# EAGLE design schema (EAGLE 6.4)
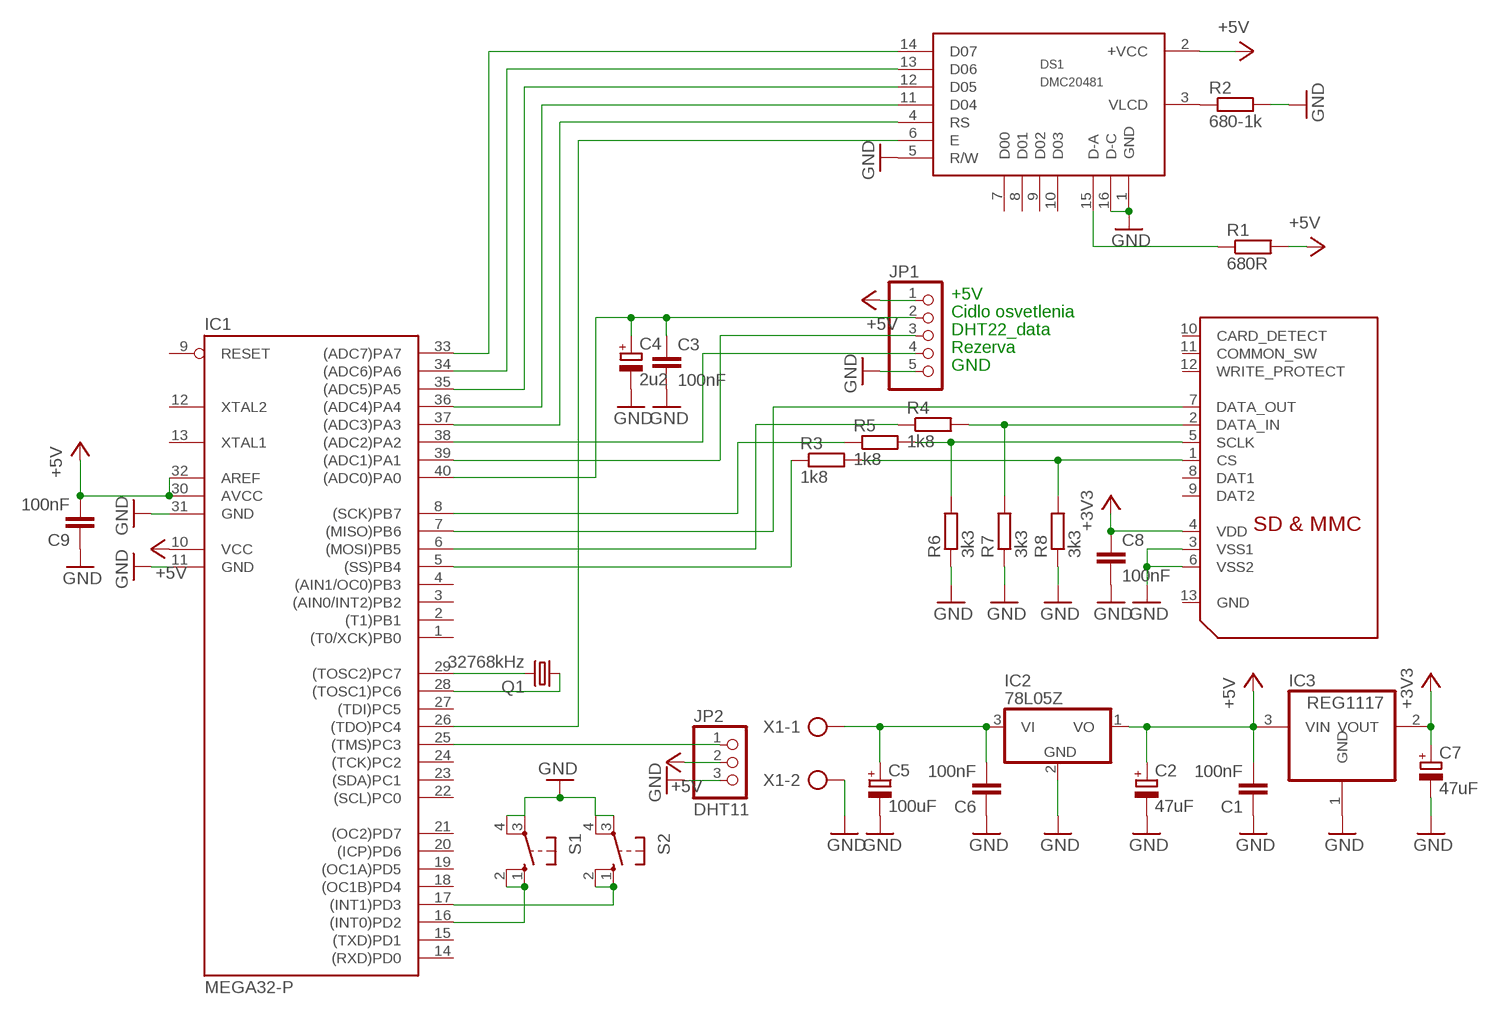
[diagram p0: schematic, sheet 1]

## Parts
C1  100nF  C-EU050-024X044  [C050-024X044]
C2  47uF  CPOL-EUE2.5-5  [E2,5-5]
C3  100nF  C-EU050-024X044  [C050-024X044]
C4  2u2  CPOL-EUE2.5-5  [E2,5-5]
C5  100uF  CPOL-EUE2.5-5  [E2,5-5]
C6  100nF  C-EU050-024X044  [C050-024X044]
C7  47uF  CPOL-EUE2.5-5  [E2,5-5]
C8  100nF  C-EU050-024X044  [C050-024X044]
C9  100nF  C-EU050-024X044  [C050-024X044]
DS1  DMC20481  [DM20481]
IC1  MEGA32-P  [DIL40]
IC2  78L05Z  [TO92]
IC3  REG1117  [SOT223]
JP1  PINHD-1X5  [1X05]
JP2  DHT11  PINHD-1X3  [1X03]
Q1  32768kHz  CRYSTALTC26V  [TC26V]
R1  680R  R-EU_0207/10  [0207/10]
R2  680-1k  R-EU_0207/10  [0207/10]
R3  1k8  R-EU_0207/10  [0207/10]
R4  1k8  R-EU_0207/10  [0207/10]
R5  1k8  R-EU_0207/10  [0207/10]
R6  3k3  R-EU_0207/10  [0207/10]
R7  3k3  R-EU_0207/10  [0207/10]
R8  3k3  R-EU_0207/10  [0207/10]
S1  10-XX  [B3F-10XX]
S2  10-XX  [B3F-10XX]
U$1  SDMMCSCDA  [SCDA]
X1  AK500/2  [AK500/2]

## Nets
+3V3: C7.+ C8.1 IC3.2(VOUT) U$1.4(VDD)
+5V: C1.2 C2.+ C9.2 DS1.2(+VCC) IC1.10(VCC) IC1.30(AVCC) IC1.32(AREF) IC2.1(VO) IC3.3(VIN) JP1.1 JP2.2 R1.2
GND: C1.1 C2.- C3.2 C4.- C5.- C6.1 C7.- C8.2 C9.1 DS1.1(GND) DS1.5(R/W) DS1.16(D-C) IC1.11(GND) IC1.31(GND) IC2.2(GND) IC3.1(GND) JP1.5 JP2.3 R2.2 R6.1 R7.1 R8.1 S1.3(P) S1.4(P1) S2.3(P) S2.4(P1) U$1.3(VSS1) U$1.6(VSS2) X1.2
N$1: IC1.28((TOSC1)PC6) Q1.1
N$2: IC1.29((TOSC2)PC7) Q1.2
N$3: C3.1 C4.+ IC1.40((ADC0)PA0) JP1.2
N$4: IC1.39((ADC1)PA1) JP1.3
N$5: IC1.38((ADC2)PA2) JP1.4
N$6: DS1.11(D04) IC1.36((ADC4)PA4)
N$7: DS1.12(D05) IC1.35((ADC5)PA5)
N$8: DS1.13(D06) IC1.34((ADC6)PA6)
N$9: DS1.14(D07) IC1.33((ADC7)PA7)
N$10: DS1.15(D-A) R1.1
N$11: DS1.3(VLCD) R2.1
N$13: DS1.4(RS) IC1.37((ADC3)PA3)
N$15: C5.+ C6.2 IC2.3(VI) X1.1
N$16: R5.2 R6.2 U$1.5(SCLK)
N$17: IC1.16((INT0)PD2) S1.1(S) S1.2(S1)
N$18: IC1.17((INT1)PD3) S2.1(S) S2.2(S1)
N$19: IC1.25((TMS)PC3) JP2.1
N$20: IC1.5((SS)PB4) R3.1
N$21: IC1.6((MOSI)PB5) R4.1
N$22: IC1.7((MISO)PB6) U$1.7(DATA_OUT)
N$23: IC1.8((SCK)PB7) R5.1
N$24: R4.2 R7.2 U$1.2(DATA_IN)
N$25: R3.2 R8.2 U$1.1(CS)
N$66: DS1.6(E) IC1.26((TDO)PC4)
Unconnected: DS1.7(D00) DS1.8(D01) DS1.9(D02) DS1.10(D03) IC1.1((T0/XCK)PB0) IC1.2((T1)PB1) IC1.3((AIN0/INT2)PB2) IC1.4((AIN1/OC0)PB3) IC1.9(RESET) IC1.12(XTAL2) IC1.13(XTAL1) IC1.14((RXD)PD0) IC1.15((TXD)PD1) IC1.18((OC1B)PD4) IC1.19((OC1A)PD5) IC1.20((ICP)PD6) IC1.21((OC2)PD7) IC1.22((SCL)PC0) IC1.23((SDA)PC1) IC1.24((TCK)PC2) IC1.27((TDI)PC5) U$1.8(DAT1) U$1.9(DAT2) U$1.10(CARD_DETECT) U$1.11(COMMON_SW) U$1.12(WRITE_PROTECT) U$1.13(GND)

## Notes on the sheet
- +5V
- Cidlo osvetlenia
- DHT22_data
- Rezerva
- GND

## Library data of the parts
C1 C3 C6 C8 C9 = rcl:C-EU: CAPACITOR, European symbol
C2 C4 C5 C7 = rcl:CPOL-EU: POLARIZED CAPACITOR, European symbol
DS1 = abi-lcd:DMC20481
IC1 = atmel:MEGA32-P: MICROCONTROLLER 32 Kbytes FLASH 2 Kbytes SRAM 1 Kbytes EEPROM USART 8-channel 10 bit ADC Source: www.atmel.com .. doc2503.pdf; MPN: ATMEGA32-16PU; OC_FARNELL: 1661729; OC_NEWARK: 51P1794
IC2 = linear:78*: Positive VOLTAGE REGULATOR Source: http://cache.national.com/ds/LM/LM78L05.pdf http://www.fairchildsemi.com/ds/LM/LM7805.pdf
IC3 = burr-brown:REG1117: 800mA and 1A Low Dropout (LDO) Positive Regulator 1.8V, 2.5V, 2.85V, 3.3V, 5V, and Adj; MPN: REG1117; OC_FARNELL: 1097566; OC_NEWARK: 14P6981
JP1 = pinhead:PINHD-1X5: PIN HEADER
JP2 = pinhead:PINHD-1X3: PIN HEADER
Q1 = crystal:CRYSTAL: CRYSTAL; OC_FARNELL: unknown; OC_NEWARK: unknown
R1-R8 = rcl:R-EU_: RESISTOR, European symbol
S1 S2 = switch-omron:10-XX: OMRON SWITCH; MPN: B3F-1000; OC_FARNELL: 176432; OC_NEWARK: 36M3542
U$1 = adafruit:SDMMC: SD MMC Card holder 4UCON part #06132 - easy to solder
X1 = con-ptr500:AK500/2: CONNECTOR; OC_FARNELL: unknown; OC_NEWARK: unknown

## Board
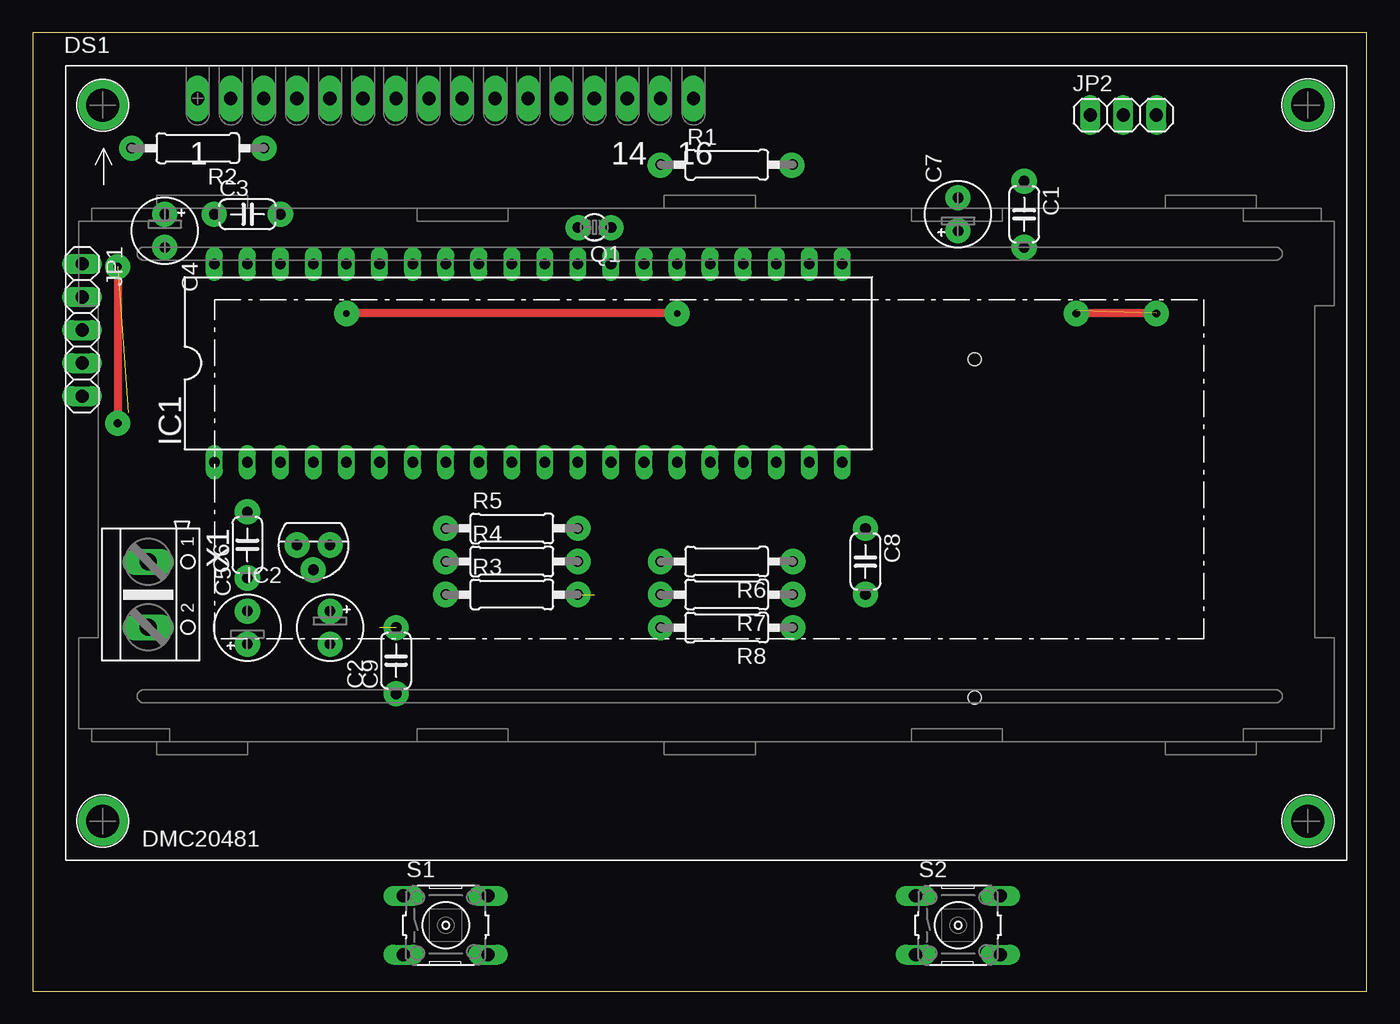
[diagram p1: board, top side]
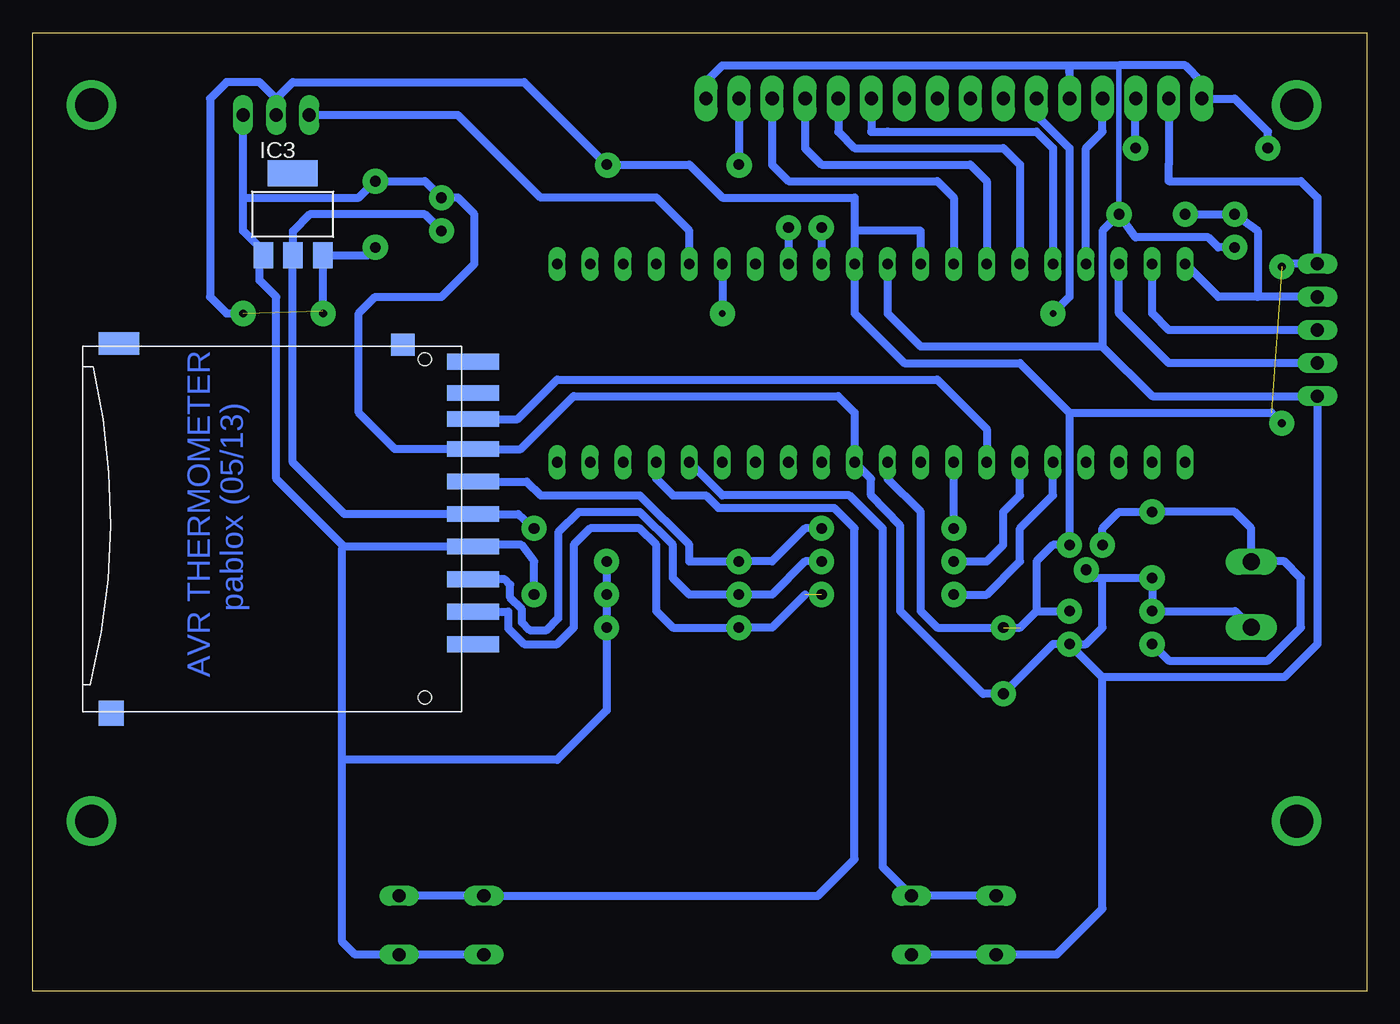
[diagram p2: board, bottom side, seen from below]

Size 102.54 x 73.65 mm. Coordinates in mm from the lower left corner, seen from the top.
Outline: 0,0 102.54,0 102.54,73.65 0,73.65 0,0
Copper layers (1*16): Top 0.035mm / dielectric 1.5mm / Bottom 0.035mm
Design rules "default": minimum track width 10mil, minimum drill 24mil, track to track 8mil, track to pad 8mil, pad to pad 8mil, via to via 8mil, smd to smd 8mil, copper to edge 40mil, drill to drill 8mil, minimum pad ring 10mil, minimum via ring 8mil, stop-mask expansion 4mil, vias tented up to drill 0mil, thermal gap 10mil

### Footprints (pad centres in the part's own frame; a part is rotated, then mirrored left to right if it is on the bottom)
C050-024X044 = drill 0.813 octagon: 1 -2.54,0; 2 2.54,0
E2,5-5 = drill 0.813 pad 1.6: + -1.27,0 | drill 0.813 pad 1.6 octagon: - 1.27,0
DM20481 = drill 1.016 pad 1.778 long: 1 -39.383,29.21; 2 -36.843,29.21; 3 -34.303,29.21; 4 -31.763,29.21; 5 -29.223,29.21; 6 -26.683,29.21; 7 -24.143,29.21; 8 -21.603,29.21; 9 -19.063,29.21; 10 -16.523,29.21; 11 -13.983,29.21; 12 -11.443,29.21; 13 -8.903,29.21; 14 -6.363,29.21; 15 -3.823,29.21; 16 -1.283,29.21 | drill 2.54 pad 3.81: P$1 -46.672,-26.289; P$2 45.936,-26.289; P$3 45.936,28.715; P$4 -46.672,28.702
DIL40 = drill 0.813 long: 1 -24.13,-7.62; 2 -21.59,-7.62; 3 -19.05,-7.62; 4 -16.51,-7.62; 5 -13.97,-7.62; 6 -11.43,-7.62; 7 -8.89,-7.62; 8 -6.35,-7.62; 9 -3.81,-7.62; 10 -1.27,-7.62; 11 1.27,-7.62; 12 3.81,-7.62; 13 6.35,-7.62; 14 8.89,-7.62; 15 11.43,-7.62; 16 13.97,-7.62; 17 16.51,-7.62; 18 19.05,-7.62; 19 21.59,-7.62; 20 24.13,-7.62; 21 24.13,7.62; 22 21.59,7.62; 23 19.05,7.62; 24 16.51,7.62; 25 13.97,7.62; 26 11.43,7.62; 27 8.89,7.62; 28 6.35,7.62; 29 3.81,7.62; 30 1.27,7.62; 31 -1.27,7.62; 32 -3.81,7.62; 33 -6.35,7.62; 34 -8.89,7.62; 35 -11.43,7.62; 36 -13.97,7.62; 37 -16.51,7.62; 38 -19.05,7.62; 39 -21.59,7.62; 40 -24.13,7.62
TO92 = drill 0.813 octagon: 1 -1.27,0; 2 0,1.905; 3 1.27,0
SOT223 = smd 1.499 x 2.007: 1 -2.261,-3.15; 2 0.025,-3.15; 3 2.311,-3.15 | smd 3.81 x 2.007: 4 0,3.15
1X05 = drill 1.016 long: 1 -5.08,0; 2 -2.54,0; 3 0,0; 4 2.54,0; 5 5.08,0
1X03 = drill 1.016 long: 1 -2.54,0; 2 0,0; 3 2.54,0
TC26V = drill 0.813: 1 -1.27,0; 2 1.27,0
0207/10 = drill 0.813 octagon: 1 -5.08,0; 2 5.08,0
B3F-10XX = drill 1.016 long: 1 -3.251,2.261; 2 3.251,2.261; 3 -3.251,-2.261; 4 3.251,-2.261
SCDA = smd 1.2 x 4: 1 6.4,3.7; 2 3.9,3.7; 3 1.4,3.7; 4 -1.1,3.7; 5 -3.6,3.7; 6 -6.1,3.7; 7 -8.4,3.7; 8 -10.4,3.7; 9 8.9,3.7; 10 -12.8,3.7 | smd 1.7 x 1.8: 11 -14.1,-1.7 | smd 1.7 x 3.1: 12 -14.2,-23.5 | smd 1.9 x 1.9: 13 14.2,-24.1 | hole 1: -13,0; 13,0
AK500/2 = drill 1.321 long: 1 -2.515,0; 2 2.515,0

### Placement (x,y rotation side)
C1  76.2,59.69 270 top
C2  22.86,27.94 270 top
C3  16.51,59.69 0 top
C4  10.16,58.42 270 top
C5  16.51,27.94 90 top
C6  16.51,34.29 90 top
C7  71.12,59.69 90 top
C8  64,33.02 270 top
C9  27.94,25.4 90 top
DS1  52.07,39.37 0 top
IC1  38.1,48.26 0 top
IC2  21.59,34.29 180 top
IC3  82.55,59.69 0 bottom
JP1  3.81,50.8 270 top
JP2  83.82,67.31 0 top
Q1  43.18,58.69 180 top
R1  53.34,63.5 0 top
R2  12.7,64.77 180 top
R3  36.83,30.48 0 top
R4  36.83,33.02 0 top
R5  36.83,35.56 0 top
R6  53.34,33.02 180 top
R7  53.34,30.48 180 top
R8  53.34,27.94 180 top
S1  31.75,5.08 0 top
S2  71.12,5.08 0 top
U$1  72.39,35.56 270 bottom
X1  8.89,30.48 270 top

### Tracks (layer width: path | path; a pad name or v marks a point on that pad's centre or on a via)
+3V3
  Bottom 0.61: C7.+ 72.39,59.69 81.23,59.69 82.53,58.4 IC3.2 82.55,56.52 82.55,40.64 78.57,36.66 U$1.4 65.2,36.66 C8.1
+5V  (3 unrouted)
  Bottom 0.61: 39.37,58.42 39.37,60.96 49.53,60.96 52.07,63.5 R1.2 64.77,69.85 82.55,69.85 83.82,68.58 | 39.37,58.42 IC1.30 39.37,52.07 35.56,48.26 26.67,48.26 22.86,44.45 | DS1.2 15.23,63.51 15.24,62.23 5.08,62.23 3.81,60.96 JP1.1 6.31,55.88 6.54,55.65 | C1.2 76.81,56.54 IC3.3 80.24,52.3 80.21,52.07 | 25.4,29.21 26.67,27.94 33.02,27.94 34.29,29.21 34.29,36.83 36.83,39.37 IC1.10 | 25.4,29.21 C2.+ | IC1.32 34.29,58.42 39.37,58.42 | 22.86,44.45 IC2.1 24.13,34.29 25.4,33.02 25.4,29.21 | 22.86,44.45 7.34,44.45 6.54,43.65 | JP2.2 83.82,68.58 | 83.82,68.58 85.09,69.85 87.63,69.85 88.9,68.58 88.9,53.34 87.63,52.07 86.36,52.07
GND
  Bottom 0.406: 19.05,71.12 C3.2
  Bottom 0.61: 22.85,69.86 DS1.5 22.85,70.84 22.84,70.85 22.84,71.1 22.86,71.12 | 22.85,69.86 22.86,71.12 | 12.7,68.59 12.7,69.85 13.97,71.12 19.05,71.12 22.86,71.12 | 12.7,68.59 DS1.1 | DS1.1 10.16,68.58 7.62,66.04 R2.2 | DS1.16 50.79,69.86 49.53,71.12 22.86,71.12 | X1.2 10.13,29.21 C5.- C6.1 20.32,31.75 | 20.32,31.75 20.95,31.75 IC2.2 | C2.- 21.59,26.67 20.32,27.94 20.32,31.75 | R7.1 R8.1 58.42,25.4 | 20.32,24.13 6.35,24.13 3.81,26.67 JP1.5 16.51,45.72 20.32,49.53 | 20.32,24.13 C2.- | U$1.3 68.69,34.18 68.58,34.29 | C4.- 11.43,57.15 12.2,57.92 17.78,57.92 C3.2 20.32,58.42 20.32,49.53 | DS1.1 12.7,68.59 | 22.85,69.86 22.86,69.85 | IC1.31 36.83,52.07 34.29,49.53 20.32,49.53 | 86.36,60.96 JP2.3 | 86.36,60.96 86.36,58.42 84.81,56.87 IC3.1 85.09,56.26 85.09,54.61 83.82,53.34 83.82,39.37 78.61,34.16 | 86.36,60.96 77.47,60.96 C1.1 72.39,62.23 C7.- 69.85,60.96 68.58,59.69 68.58,55.88 71.12,53.34 76.2,53.34 77.47,52.07 77.47,44.45 74.68,41.66 U$1.6 65.02,41.66 60.96,45.72 40.64,45.72 39.37,44.45 IC1.11 38.1,39.37 38.1,38.1 35.86,35.76 35.86,29.21 29.51,22.86 C9.1 24.13,26.67 C2.- | 20.32,24.13 20.32,6.35 23.85,2.82 S1.3 S1.4 | U$1.3 78.61,34.16 | R6.1 R7.1 | C8.2 64,33.02 64.97,34.29 68.56,34.29 U$1.3 | S2.3 S2.4 77.75,2.82 78.74,3.81 78.74,17.78 | 78.74,17.78 62.23,17.78 58.42,21.59 R7.1 | 78.74,17.78 78.74,34.03 78.61,34.16
N$1
  Bottom 0.61: Q1.1 IC1.28
N$2
  Bottom 0.61: Q1.2 IC1.29
N$3
  Bottom 0.61: JP1.2 8.39,53.34 | 8.39,53.34 11.43,53.34 IC1.40 | C3.1 C4.+ 8.39,58.42 8.39,53.34
N$4
  Bottom 0.61: JP1.3 15.24,50.8 16.51,52.07 IC1.39
N$5
  Bottom 0.61: JP1.4 15.24,48.26 19.05,52.07 IC1.38
N$6
  Bottom 0.61: DS1.11 38.09,66.05 | 38.09,66.05 38.1,66.04 | 38.09,66.05 38.09,66.03 36.83,66.04 25.4,66.04 24.13,64.77 IC1.36
N$7
  Bottom 0.61: DS1.12 40.63,66.03 39.37,64.77 27.94,64.77 26.67,63.5 IC1.35
N$8
  Bottom 0.61: DS1.13 43.17,64.76 41.91,63.5 30.48,63.5 29.21,62.23 IC1.34
N$9
  Bottom 0.61: DS1.14 45.71,63.49 44.45,62.23 33.02,62.23 31.75,60.96 IC1.33
N$10
  Bottom 0.61: DS1.15 48.25,63.51 R1.1
N$11
  Bottom 0.61: R2.1 17.78,68.57 DS1.3
N$12  (via drill 0.6 pad 1.93)
  Top 0.61: v6.54,55.65 v6.54,43.65
N$13
  Bottom 0.61: IC1.37 21.59,64.77 20.32,66.04 20.32,68.57 DS1.4
N$15
  Bottom 0.61: IC2.3 20.32,35.56 19.05,36.83 C6.2 10.16,36.83 8.89,35.56 X1.1 8.87,33.02 6.35,33.02 5.08,31.75 5.08,27.94 7.62,25.4 15.24,25.4 C5.+
N$16
  Bottom 0.61: U$1.5 64.56,39.16 63.5,38.1 55.88,38.1 52.07,34.29 52.07,33.02 R6.2 45.72,33.02 43.18,35.56 R5.2
N$17
  Bottom 0.61: S1.1 S1.2 37.23,9.57 37.23,35.56 39.77,38.1 49.53,38.1 IC1.16
N$18
  Bottom 0.61: IC1.17 54.61,39.37 53.34,38.1 50.8,38.1 49.83,37.13 40.94,37.13 39.37,35.56 39.37,10.16 42.19,7.34 S2.1 S2.2
N$19
  Bottom 0.61: IC1.25 52.07,58.42 54.61,60.96 63.5,60.96 69.85,67.31 JP2.1
N$20
  Bottom 0.61: R3.1 29.21,30.48 26.67,33.02 26.67,35.56 24.13,38.1 IC1.5
N$21
  Bottom 0.61: R4.1 29.21,33.02 27.94,34.29 27.94,36.83 26.67,38.1 IC1.6
N$22
  Bottom 0.61: IC1.7 29.21,43.18 33.02,46.99 62.23,46.99 65.26,43.96 U$1.7
N$23
  Bottom 0.61: R5.1 IC1.8
N$24
  Bottom 0.61: R4.2 43.18,33.02 45.72,30.48 R7.2 52.07,30.48 53.34,31.75 53.34,34.29 55.88,36.83 60.56,36.83 62.14,35.25 62.14,28.65 63.04,27.75 64.34,27.75 64.94,28.35 64.94,29.35 65.84,30.25 65.84,31.25 66.24,31.65 U$1.2
N$25  (1 unrouted)
  Bottom 0.61: 43.18,30.48 45.72,27.94 R8.2 53.34,27.94 54.61,29.21 54.61,34.29 55.88,35.56 59.69,35.56 60.96,34.29 60.96,27.94 62.23,26.67 64.77,26.67 65.99,27.89 65.99,29.16 U$1.1
N$26  (via drill 0.5 pad 1.93)
  other vias: 27.94,22.86
N$27  (via drill 0.6 pad 1.93)
  Top 0.61: v86.36,52.07 v80.21,52.07
N$28  (via drill 0.5 pad 1.93)
  other vias: 27.94,27.94
N$29  (via drill 0.6 pad 1.93)
  other vias: 19.05,59.69
N$30  (via drill 0.6 pad 1.93)
  other vias: 13.97,59.69
N$31  (via drill 0.6 pad 1.93)
  other vias: 17.78,64.77
N$32  (via drill 0.6 pad 1.93)
  other vias: 7.62,64.77
N$33  (via drill 0.6 pad 1.93)
  other vias: 48.24,63.45
N$34  (via drill 0.6 pad 1.93)
  other vias: 41.94,58.65
N$35  (via drill 0.6 pad 1.93)
  other vias: 44.44,58.65
N$36  (via drill 0.6 pad 1.93)
  other vias: 58.34,63.45
N$37  (via drill 0.6 pad 1.93)
  other vias: 76.2,62.23
N$38  (via drill 0.6 pad 1.93)
  other vias: 76.2,57.15
N$39  (via drill 0.6 pad 1.93)
  other vias: 48.26,30.48
N$40  (via drill 0.6 pad 1.93)
  other vias: 31.75,33.02
N$41  (via drill 0.6 pad 1.93)
  other vias: 31.75,30.48
N$42  (via drill 0.6 pad 1.93)
  other vias: 41.91,35.56
N$43  (via drill 0.6 pad 1.93)
  other vias: 41.91,33.02
N$44  (via drill 0.6 pad 1.93)
  other vias: 48.26,27.94
N$45  (via drill 0.6 pad 1.93)
  other vias: 58.42,33.02
N$46  (via drill 0.6 pad 1.93)
  other vias: 48.26,33.02
N$47  (via drill 0.6 pad 1.93)
  other vias: 41.91,30.48
N$48  (via drill 0.6 pad 1.93)
  other vias: 31.75,35.56
N$49  (via drill 0.6 pad 1.93)
  other vias: 58.42,30.48
N$50  (via drill 0.6 pad 1.93)
  other vias: 58.42,27.94
N$51  (via drill 0.6 pad 1.93)
  other vias: 20.32,34.29
N$52  (via drill 0.6 pad 1.93)
  other vias: 22.86,34.29
N$53  (via drill 0.6 pad 1.93)
  other vias: 21.57,32.37
N$54  (via drill 0.6 pad 1.93)
  other vias: 16.51,31.75
N$55  (via drill 0.6 pad 1.93)
  other vias: 16.51,29.21
N$56  (via drill 0.6 pad 1.93)
  other vias: 16.51,36.83
N$57  (via drill 0.6 pad 1.93)
  other vias: 22.86,26.67
N$58  (via drill 0.6 pad 1.93)
  other vias: 22.86,29.21
N$59  (via drill 0.6 pad 1.93)
  other vias: 16.51,26.67
N$60  (via drill 0.6 pad 1.93)
  other vias: 71.12,58.42
N$61  (via drill 0.6 pad 1.93)
  other vias: 71.12,60.96
N$62  (via drill 0.6 pad 1.93)
  other vias: 10.16,57.15
N$63  (via drill 0.6 pad 1.93)
  other vias: 10.16,59.69
N$64  (via drill 0.5 pad 1.93)
  other vias: 64,35.56
N$65  (via drill 0.5 pad 1.93)
  other vias: 64,30.48
N$66  (via drill 0.5 pad 1.93)
  Top 0.61: v49.53,52.07 v24.13,52.07
  Bottom 0.61: DS1.6 25.39,67.3 22.86,64.77 22.86,53.34 v24.13,52.07 | IC1.26 v49.53,52.07

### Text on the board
Bottom: pablox (05/13) | AVR THERMOMETER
